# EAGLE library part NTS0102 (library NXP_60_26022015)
Dual supply translating transceiver; open drain; auto direction sensing
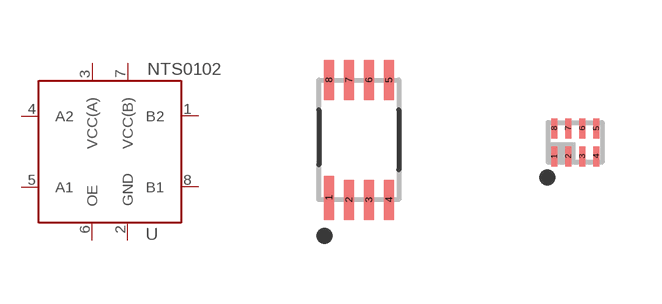
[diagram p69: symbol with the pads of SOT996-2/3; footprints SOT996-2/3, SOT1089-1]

Designator prefix U

## NTS0102GD  [SOT996-2/3]
1  B2  out
2  GND  out
3  VCC(A)  out
4  A2  out
5  A1  out
6  OE  out
7  VCC(B)  out
8  B1  out

## NTS0102GF  [SOT1089-1]
Pads as for SOT996-2/3

## NTS0102GU  [SOT1160-1]
1  A2  out
2  VCC(A)  out
4  OE  out
5  B2  out
6  VCC(B)  out
8  B1  out
9  GND  out
10  A1  out

## NTS0102DP  [SOT505-2]
Pads as for SOT996-2/3

## Footprint SOT996-2/3 (pad centres in mm)
SOT996-2/3 XSON8U: plastic extremely thin small outline package; no leads;8 terminals; UTLP based; body 3 x 2 x 0.5 mm JEDEC: IEC: -- JEITA: --
smd 0.25 x 1.1: 1 -0.75,-1.45
smd 0.25 x 1: 2 -0.25,-1.5; 3 0.25,-1.5; 4 0.75,-1.5; 5 0.75,1.5; 6 0.25,1.5; 7 -0.25,1.5; 8 -0.75,1.5

## Footprint SOT1089-1 (pad centres in mm)
SOT1089-1 XSON8: plastic, extremely thin small outline package; no leads; 8 terminals; body 1 x 1.35 x 0.5 mm JEDEC: -- IEC: -- JEITA: --
smd 0.15 x 0.5: 1 -0.525,-0.35; 2 -0.175,-0.35; 3 0.175,-0.35; 4 0.525,-0.35; 5 0.525,0.35; 6 0.175,0.35; 7 -0.175,0.35; 8 -0.525,0.35

## Footprint SOT1160-1 (pad centres in mm)
SOT1160-1 XQFN10: plastic, extremely thin quad flat package; no leads;10 terminals; body 1.40 x 1.80 x 0.50 mm JEDEC: -- IEC: -- JEITA: --
smd 0.65 x 0.22: 1 -0.525,0.2
smd 0.55 x 0.22: 2 -0.575,-0.2; 6 0.575,-0.2; 7 0.575,0.2
smd 0.22 x 0.55: 3 -0.4,-1; 4 0,-1; 5 0.4,-1; 8 0.4,1; 9 0,1; 10 -0.4,1

## Footprint SOT505-2 (pad centres in mm)
SOT505-2 TSSOP8: plastic thin shrink small outline package; 8 leads; body width 3 mm JEDEC: -- IEC: --
smd 0.5 x 0.85: 1 -1.025,-1.775; 4 1.025,-1.775; 5 1.025,1.775; 8 -1.025,1.775
smd 0.4 x 0.85: 2 -0.325,-1.775; 3 0.325,-1.775; 6 0.325,1.775; 7 -0.325,1.775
